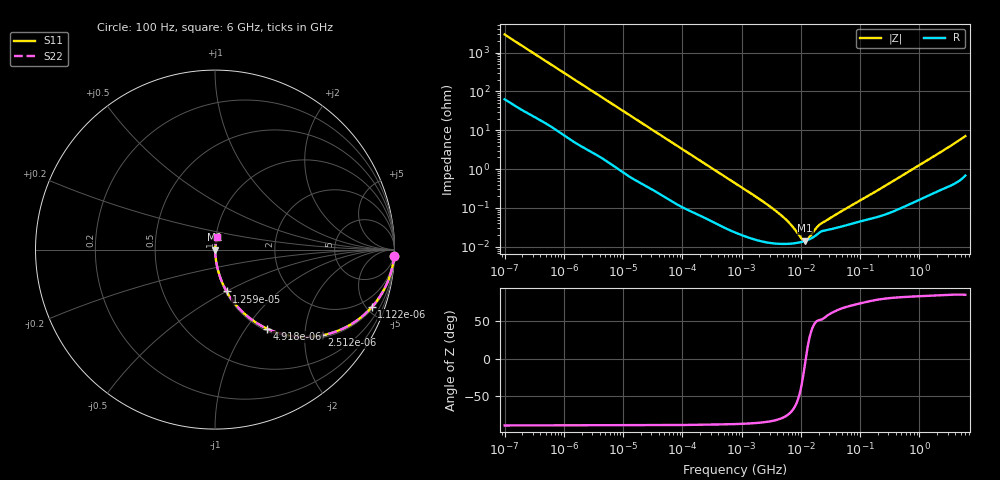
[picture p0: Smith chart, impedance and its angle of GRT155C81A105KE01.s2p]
!Murata Part Number: GRT155C81A105KE01
!These Parameters are Measured in Series Mode Connection
!Data Generated on Jun 19, 2026
!  o--ll--o
!Port1  Port2
!  o------o
!Operation Temp=25[degC], DC Bias Voltage=0[V]
!Freq. Start=100[Hz] Stop=6[GHz] 401[Steps]
# Hz S RI R 50
!Freq.(Hz) S11(Real) S11(Imag) S21(Real) S21(Imag) S12(Real) S12(Imag) S22(Real) S22(Imag)
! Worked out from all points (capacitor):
!   401 points, 100 Hz to 6 GHz, reference 50 ohm
!   read as one part in series: C = 542 nF near 109 Hz
!   lowest |Z| = 14.3 mohm at 11.89 MHz (marker M1)
!   series resonance near 12.14 MHz, so ESL is about 320 pH
!   S11 on the Smith chart (normalised r, x): 100 Hz: 2, -58; 1.122 kHz: 1.13, -5.41; 2.512 kHz: 1.06, -2.44; 4.918 kHz: 1.03, -1.26; 12.59 kHz: 1.01, -0.50; 6 GHz: 1.01, +0.14
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100  0.9981 -0.0341  0.0019 0.0341  0.0019 0.0341  0.9981 -0.0341
383  0.9808 -0.1256  0.0192 0.1256  0.0192 0.1256  0.9808 -0.1256
1122  0.8739 -0.32  0.1261 0.32  0.1261 0.32  0.8739 -0.32
2008  0.6946 -0.4483  0.3054 0.4483  0.3054 0.4483  0.6946 -0.4483
2512  0.5967 -0.4779  0.4033 0.4779  0.4033 0.4779  0.5967 -0.4779
3437  0.4481 -0.4841  0.5519 0.4841  0.5519 0.4841  0.4481 -0.4841
4918  0.2908 -0.4407  0.7092 0.4407  0.7092 0.4407  0.2908 -0.4407
7695  0.1488 -0.343  0.8512 0.343  0.8512 0.343  0.1488 -0.343
12592  0.0645 -0.233  0.9355 0.233  0.9355 0.233  0.0645 -0.233
40335  0.00863 -0.0789  0.9914 0.0789  0.9914 0.0789  0.00863 -0.0789
129199  0.00151 -0.0254  0.9985 0.0254  0.9985 0.0254  0.00151 -0.0254
774597  0.000254 -0.00439  0.9997 0.00439  0.9997 0.00439  0.000254 -0.00439
4246196  0.00012 -0.000723  0.9999 0.000723  0.9999 0.000723  0.00012 -0.000723
6644369  0.000121 -0.000368  0.9999 0.000368  0.9999 0.000368  0.000121 -0.000368
1.039699e7  0.000134 -8.89e-05  0.9999 8.89e-05  0.9999 8.89e-05  0.000134 -8.89e-05
1.189169e7  0.000142 -1.16e-05  0.9999 1.16e-05  0.9999 1.16e-05  0.000142 -1.16e-05
1.300572e7  0.00015 3.95e-05  0.9999 -3.95e-05  0.9999 -3.95e-05  0.00015 3.95e-05
1.555665e7  0.00017 0.000141  0.9998 -0.000141  0.9998 -0.000141  0.00017 0.000141
1.86079e7  0.000206 0.00024  0.9998 -0.00024  0.9998 -0.00024  0.000206 0.00024
2.225763e7  0.00025 0.000316  0.9997 -0.000316  0.9997 -0.000316  0.00025 0.000316
3.124326e8  0.000761 0.00425  0.9992 -0.00425  0.9992 -0.00425  0.000761 0.00425
6e9  0.0116 0.0692  0.9884 -0.0692  0.9884 -0.0692  0.0116 0.0692
